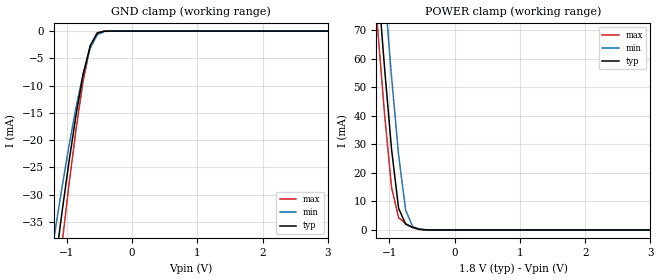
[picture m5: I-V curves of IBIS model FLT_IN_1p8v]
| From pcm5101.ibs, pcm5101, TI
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|   FLT_IN_1p8v
[Model]   FLT_IN_1p8v
Model_type   Input
Vinl = 0.54
Vinh = 1.26
|   typ   min   max
C_comp   1.492329547pF   1.472260021pF   1.515772755pF
[Voltage Range]   1.8   1.65   1.95
[Temperature Range]   27   105   -25
[Power Clamp Reference]   1.8   1.65   1.95
[GND Clamp Reference]   -0   -0   -0
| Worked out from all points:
|   GND clamp passes 1 mA (typ) near -0.56 V on its own axis
|   POWER clamp passes 1 mA (typ) near -0.66 V on its own axis
[GND Clamp]
|   Voltage   I(typ)   I(min)   I(max)
-1.8V     -105.9mA   -88.79mA   -122.2mA
-1.182V   -43.15mA   -36.82mA   -50.61mA
-1.074V   -33.22mA   -28.66mA   -39.05mA
-966.5mV  -23.87mA   -20.97mA   -28.07mA
-858.5mV  -15.31mA   -13.91mA   -17.93mA
-750.5mV  -7.963mA   -7.777mA   -9.142mA
-642.5mV  -2.664mA   -3.129mA   -2.804mA
-534.5mV  -378.4uA   -687.8uA   -300.4uA
-426.5mV  -22.54uA   -76.81uA   -10.61uA
-318.5mV  -722.7nA   -5.54uA    -151.4nA
3.6V      0A         0A         0A
[POWER Clamp]
|   Voltage   I(typ)   I(min)   I(max)
-1.8V     283.3mA    311.2mA    266.4mA
-1.182V   88.62mA    116.6mA    71.64mA
-1.074V   57.01mA    84.37mA    40.75mA
-966.5mV  28.23mA    53.67mA    14.9mA
-858.5mV  7.578mA    26.2mA     4.28mA
-750.5mV  2.019mA    6.936mA    2.253mA
-642.5mV  840.3uA    1.18mA     932.9uA
-534.5mV  214uA      297.3uA    193.5uA
-426.5mV  21.46uA    49.86uA    12.56uA
3.6V      0A         0A         0A
